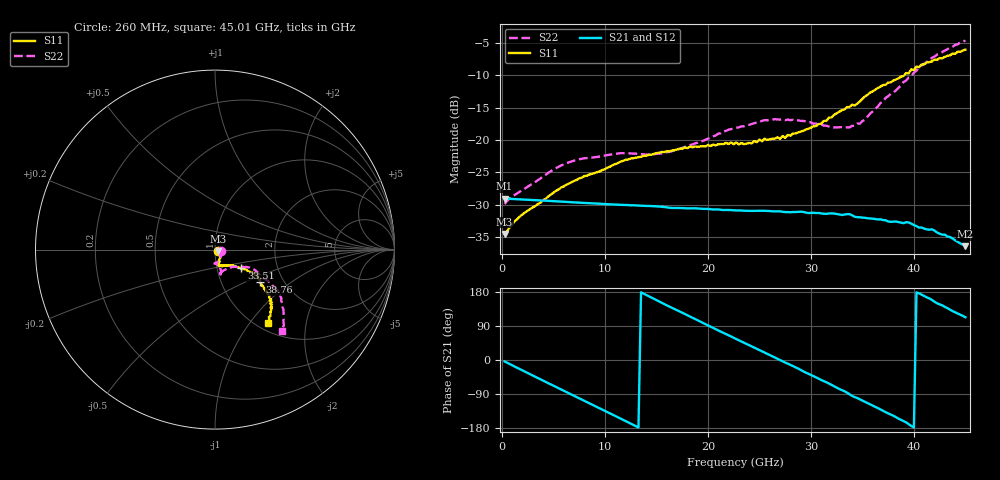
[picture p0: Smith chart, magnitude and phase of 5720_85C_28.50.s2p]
! Device:  ADRF5720
! Description: 0.5dB LSB GaAs MMIC 6-bit Digital Attenuator
! Frequency:  0.000009 -  40 GHz
! Ports:
!	RF1	= Port 1
!	RF2	= Port 2
! Vdd:  3.3 Volt
! Vss:  -3.3 Volt
! Control:  0/3.3 Volt
! State:  28.50 dB attenuation
! Data:  The device was measured using G-S-G Probes on a matrix board.
!  Data was collected using an calibrated 4 port network analyzer.
!  The reference plane for this measurement is at the launchers.
! Note:  Analog Devices supplies this data as a sample of measured data
!  for this product.  Your particular data for this product may vary.
!  Data was taken at 85 degrees C.
!  Analog Devices reserves the right to change this data at anytime.
# GHZ S DB R 45.0
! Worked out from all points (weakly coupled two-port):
!   180 points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, 260 MHz to 45.01 GHz, reference 45 ohm
!   highest |S21| = -29.07 dB at 260 MHz (marker M1); lowest = -36.5 dB at 45.01 GHz (marker M2)
!   lowest |S11| = -34.6 dB at 260 MHz (marker M3), VSWR 1.04, Z = 46.6 - j0.716 ohm
!   |S11| at or under -10 dB: start of sweep to 39.06 GHz
!   |S22| runs from -29.9 to -4.6 dB; largest |S21 - S12| = 0.00025
!   S11 on the Smith chart (normalised r, x): 260 MHz: 1.03, -0.02; 33.51 GHz: 1.31, -0.28; 38.76 GHz: 1.52, -0.61; 45.01 GHz: 1.13, -1.22
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0.26  -34.58 -24.3  -29.07 -3.7  -29.07 -3.7  -29.92 -15.9
1.26  -32.55 -1.3  -29.16 -17.6  -29.15 -17.6  -28.49 -13.1
2.26  -31.21 -9.4  -29.24 -31.2  -29.23 -31.1  -27.49 -26.8
5.26  -27.86 -42.4  -29.51 -71.3  -29.49 -71.2  -24.35 -65.4
7.76  -25.85 -54.7  -29.73 -104.5  -29.71 -104.5  -22.92 -80.5
12.01  -23.07 -69.8  -30.07 -161.1  -30.06 -161.0  -22.04 -91.9
15.26  -21.99 -76.0  -30.31 154.6  -30.30 154.7  -22.11 -87.4
17.26  -21.35 -78.8  -30.54 128.2  -30.52 128.3  -21.39 -81.9
22.76  -20.39 -72.5  -30.91 55.3  -30.89 55.5  -18.12 -74.3
23.51  -20.65 -72.0  -30.96 45.6  -30.94 45.8  -17.88 -74.5
26.51  -19.81 -60.9  -31.05 6.6  -31.04 6.8  -16.78 -76.9
27.51  -19.67 -57.2  -31.17 -6.7  -31.17 -6.4  -16.94 -77.4
30.26  -17.89 -45.6  -31.28 -42.5  -31.27 -42.3  -17.50 -77.2
33.51  -14.92 -35.6  -31.49 -86.1  -31.48 -85.8  -18.04 -56.7
34.76  -14.03 -33.8  -31.97 -103.8  -31.96 -103.5  -17.48 -45.6
35.76  -12.66 -32.6  -32.16 -117.0  -32.15 -116.7  -15.91 -37.8
37.76  -11.09 -32.1  -32.68 -144.1  -32.67 -143.7  -12.86 -27.5
38.76  -10.18 -35.8  -32.82 -157.9  -32.79 -157.3  -11.54 -28.0
40.26  -8.64 -39.1  -33.35 178.4  -33.33 178.9  -9.26 -30.7
41.76  -7.84 -41.7  -33.84 158.5  -33.79 158.6  -7.28 -34.0
43.51  -6.90 -45.5  -35.03 133.0  -35.00 133.4  -5.68 -42.7
45.01  -6.01 -54.2  -36.45 112.9  -36.43 113.5  -4.59 -50.4
